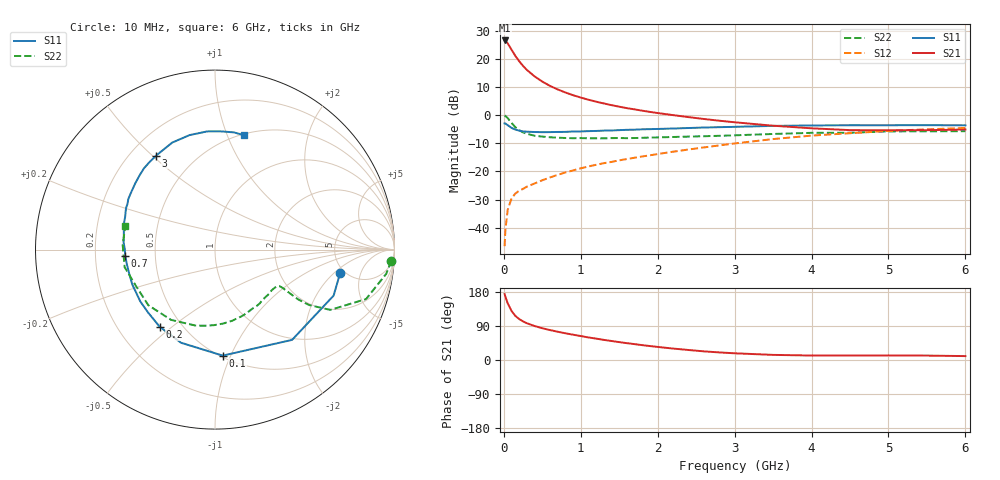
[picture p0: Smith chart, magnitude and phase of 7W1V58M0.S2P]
! Infineon Technologies  Discrete & RF Semiconductors
! BFS17W
! Si NPN RF Bipolar Junction Transistor in SOT323
! VCE = 1.5 V  IC = 8 mA
! Common Emitter S-Parameters:  August  1999
# GHz  S  MA  R  50
!  f  S11  S21  S12  S22
! GHz  MAG  ANG  MAG  ANG  MAG  ANG  MAG  ANG
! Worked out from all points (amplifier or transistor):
!   36 points, 10 MHz to 6 GHz, reference 50 ohm
!   highest |S21| = 26.5 dB at 10 MHz (marker M1)
!   |S21| within 3 dB of that: start of sweep to 93.69 MHz
!   unconditionally stable (mu >= 1): 403.8 MHz to end of sweep
!   at 250 MHz: K = 0.76, MSG = 21.8 dB, |S12| = -26.2 dB
!   at 1.4 GHz: K = 1.28, MAG = 6.9 dB, |S12| = -16.6 dB
!   at 6 GHz: K = 1.10, MAG = -2.2 dB, |S12| = -4.6 dB
!   S11 on the Smith chart (normalised r, x): 10 MHz: 4.59, -2.39; 100 MHz: 0.51, -0.93; 200 MHz: 0.38, -0.45; 700 MHz: 0.33, -0.03; 3 GHz: 0.30, +0.51; 6 GHz: 0.51, +1.15
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0.01  0.7095 -10.5  21.12 174.0  0.0047 83.0  0.9844 -3.6
0.02  0.7088 -21.2  20.93 167.1  0.0091 79.9  0.964 -8.0
0.05  0.6614 -49.5  18.76 149.7  0.0207 69.5  0.8858 -18.1
0.1  0.5922 -85.8  14.47 129.4  0.0332 55.7  0.7254 -27.6
0.15  0.5524 -110.1  11.23 116.3  0.0405 50.6  0.6088 -30.5
0.2  0.529 -125.6  9.005 108.0  0.0454 49.2  0.5385 -30.9
0.25  0.5117 -136.8  7.44 101.8  0.049 48.9  0.4923 -30.4
0.3  0.5067 -145.2  6.322 97.0  0.0535 50.1  0.4648 -30.0
0.4  0.5002 -157.2  4.854 89.6  0.061 52.5  0.4298 -29.5
0.5  0.4966 -165.2  3.93 83.9  0.0696 54.4  0.4149 -29.5
0.6  0.498 -171.2  3.295 79.0  0.0781 56.6  0.4035 -30.4
0.7  0.5015 -176.2  2.853 74.6  0.0868 58.5  0.3965 -32.0
0.9  0.5108 175.6  2.252 66.8  0.1039 60.0  0.3884 -36.1
1.1  0.5183 168.6  1.871 59.5  0.1222 60.9  0.3874 -41.3
1.3  0.5297 162.5  1.607 53.1  0.1399 61.6  0.3859 -47.2
1.6  0.5475 154.7  1.327 44.4  0.1657 61.9  0.389 -56.4
2.2  0.5771 140.5  0.998 30.2  0.2236 61.8  0.4081 -76.7
3  0.618 122.0  0.745 17.7  0.3135 57.8  0.437 -104.4
3.5  0.6422 111.8  0.647 13.5  0.3747 53.3  0.4617 -122.0
4.5  0.66 93.7  0.54 11.7  0.4759 41.1  0.4852 -155.8
5.5  0.6614 80.9  0.539 11.6  0.5578 29.4  0.515 177.1
6  0.6578 76.0  0.554 10.3  0.5903 23.9  0.517 165.2
